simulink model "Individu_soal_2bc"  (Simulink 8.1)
settings: Solver=ode45  StartTime=0.0  StopTime=3.0  RelTol=1e-3

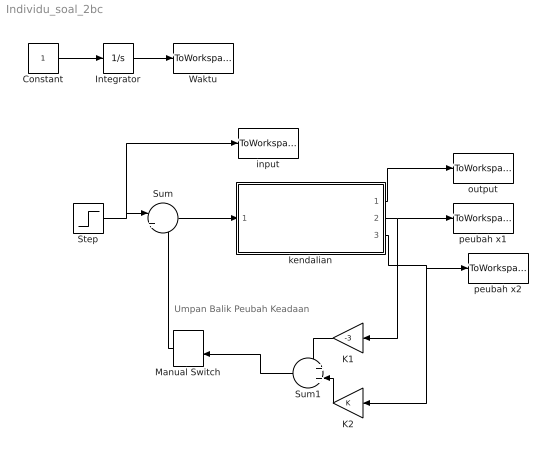
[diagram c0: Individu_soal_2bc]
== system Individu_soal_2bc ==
  note: Umpan Balik Peubah Keadaan
  Constant : Constant
  Integrator : Integrator
  K1 : Gain  Gain=-3
  K2 : Gain
  Manual Switch : ManualSwitch  CurrentSetting=0
  Step : Step  SampleTime=0
  Sum : Sum  Inputs=|+-
  Sum1 : Sum
  Waktu : ToWorkspace  VariableName=time  SampleTime=-1
  input : ToWorkspace  VariableName=u  SampleTime=-1
  kendalian : Subsystem
  output : ToWorkspace  VariableName=y  SampleTime=-1
  peubah x1 : ToWorkspace  VariableName=x1  SampleTime=-1
  peubah x2 : ToWorkspace  VariableName=x2  SampleTime=-1
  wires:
  Constant/1 -> Integrator/1
  Integrator/1 -> Waktu/1
  kendalian/1(y) -> output/1
  Step/1 -> Sum/1, input/1
  kendalian/2(x1) -> K1/1, peubah x1/1
  kendalian/3(x2) -> K2/1, peubah x2/1
  K1/1 -> Sum1/1
  K2/1 -> Sum1/2
  Sum/1 -> kendalian/1(u)
  Sum1/1 -> Manual Switch/2
  Manual Switch/1 -> Sum/2

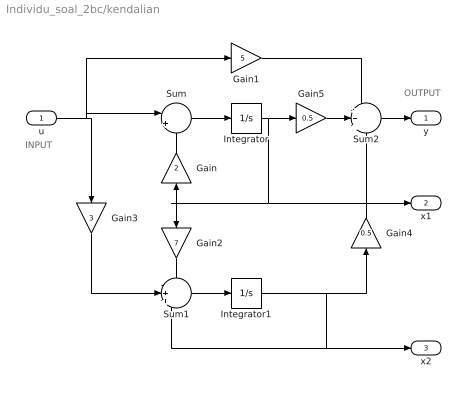
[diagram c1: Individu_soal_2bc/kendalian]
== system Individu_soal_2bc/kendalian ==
  note: INPUT
  note: OUTPUT
  u : Inport
  Gain : Gain  Gain=2
  Gain1 : Gain  Gain=5
  Gain2 : Gain  Gain=7
  Gain3 : Gain  Gain=3
  Gain4 : Gain  Gain=0.5
  Gain5 : Gain  Gain=0.5
  Integrator : Integrator
  Integrator1 : Integrator
  Sum : Sum  Inputs=|+-
  Sum1 : Sum  Inputs=-++
  Sum2 : Sum  Inputs=+++
  y : Outport
  x1 : Outport  Port=2
  x2 : Outport  Port=3
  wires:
  Integrator/1 -> Gain5/1, x1/1, Gain/1, Gain2/1
  Integrator1/1 -> Gain4/1, x2/1, Sum1/3
  u/1 -> Gain3/1, Sum/1, Gain1/1
  Sum/1 -> Integrator/1
  Sum1/1 -> Integrator1/1
  Sum2/1 -> y/1
  Gain1/1 -> Sum2/1
  Gain/1 -> Sum/2
  Gain2/1 -> Sum1/1
  Gain4/1 -> Sum2/3
  Gain3/1 -> Sum1/2
  Gain5/1 -> Sum2/2
